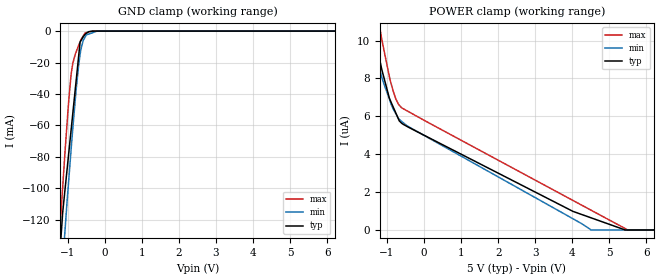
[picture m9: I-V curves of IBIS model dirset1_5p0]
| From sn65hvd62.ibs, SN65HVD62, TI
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|   dirset1_5p0 Model
[Model]   dirset1_5p0
Model_type   Input
Vinl = 1.5
Vinh = 3.5
|   typ   min   max
|   (nom PVT)   (fast PVT)   (slow PVT)
 C_comp   2.118e-12   2.012e-12   2.287e-12
| Where nom  PVT is Nominal Process, 5V, 27C
|   Fast PVT is Strong Process,  5.5V, -40C
|   Slow PVT is Weak Process,   4.5V, 125C
[Voltage Range]   5   4.5   5.5
|Ambient Temperature   25   85   -40
|Junction Temperature
[Temperature Range]   27   125   -40
[Power Clamp Reference]   5   4.5   5.5
[GND Clamp Reference]   0   0   0
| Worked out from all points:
|   GND clamp passes 1 mA (typ) near -0.47 V on its own axis
[GND Clamp]
|   Voltage   I(typ)   I(min)   I(max)
-5V       -1.641A    -1.575A    -1.709A
-1.21V    -139.8mA   -170.8mA   -124.7mA
-1.14V    -115.6mA   -147.8mA   -99.57mA
-1.078V   -101.3mA   -127.3mA   -77.32mA
-984.5mV  -79.66mA   -97.4mA    -46.65mA
-918.5mV  -64.42mA   -77.31mA   -29.07mA
-869mV    -52.99mA   -62.74mA   -20.83mA
-774mV    -31.06mA   -36.73mA   -13.14mA
-670mV    -7.045mA   -14.92mA   -6.777mA
-528mV    -1.891mA   -3.545mA   -1.101mA
-211.5mV  -17.16uA   -15.21uA   -3.643uA
10V       0A         0A         0A
[POWER Clamp]
|   Voltage   I(typ)   I(min)   I(max)
-5V       28.08uA    20.8uA     39.66uA
-1.521V   12.13uA    10.75uA    14.7uA
-1.373V   10.56uA    9.694uA    12.76uA
-1.14V    8.454uA    8.053uA    10.04uA
-935mV    6.942uA    6.895uA    8.076uA
-841.5mV  6.524uA    6.413uA    7.375uA
-693mV    5.861uA    5.894uA    6.64uA
-605mV    5.634uA    5.732uA    6.447uA
4.02V     980.3nA    589.6nA    1.557uA
4.505V    643.5nA    0A         1.047uA
5.495V    0A         0A         0A
10V       0A         0A         0A
